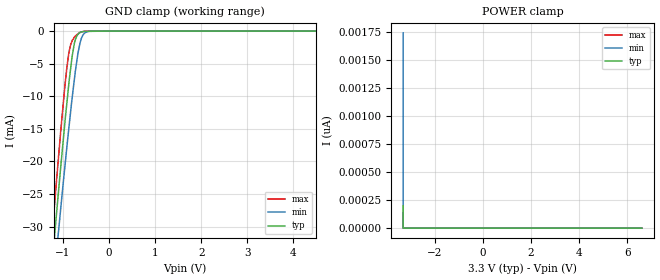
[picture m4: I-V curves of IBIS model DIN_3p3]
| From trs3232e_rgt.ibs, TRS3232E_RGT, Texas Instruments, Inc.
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[Model]   DIN_3p3
Model_type   Input
Vinl = 0.8
Vinh = 2.0
|   typ   min   max
C_comp   0.80pF   0.77pF   0.84pF
[Voltage Range]   3.3   3   3.6
[Temperature Range]   27   110   -40
[Power Clamp Reference]   3.3   3   3.6
[GND Clamp Reference]   0   0   0
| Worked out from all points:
|   GND clamp passes 1 mA (typ) near -0.71 V on its own axis
[GND Clamp]
|   Voltage   I(typ)   I(min)   I(max)
-3.3V     -208.9mA   -199.9mA   -218.1mA
-1.249V   -36.59mA   -41.76mA   -32.16mA
-1.188V   -31.75mA   -37.27mA   -26.96mA
-1.15V    -28.66mA   -34.48mA   -23.64mA
-1.051V   -20.9mA    -27.29mA   -15.42mA
-962.6mV  -14.25mA   -20.98mA   -8.635mA
-879mV    -8.425mA   -15.25mA   -3.604mA
-756.1mV  -1.97mA    -7.529mA   -967.5uA
-631.4mV  -227.7uA   -1.828mA   -207.9uA
-547.4mV  -50.67uA   -412.4uA   -55.6uA
-430.7mV  -39.29uA   -32.69uA   -11.7uA
6.6V      0A         0A         0A
[POWER Clamp]
|   Voltage   I(typ)   I(min)   I(max)
-3.3V     199.5pA    1.746nA    133.2pA
-3.3V     0A         0A         0A
-3.3V     0A         0A         0A
6.6V      0A         0A         0A
